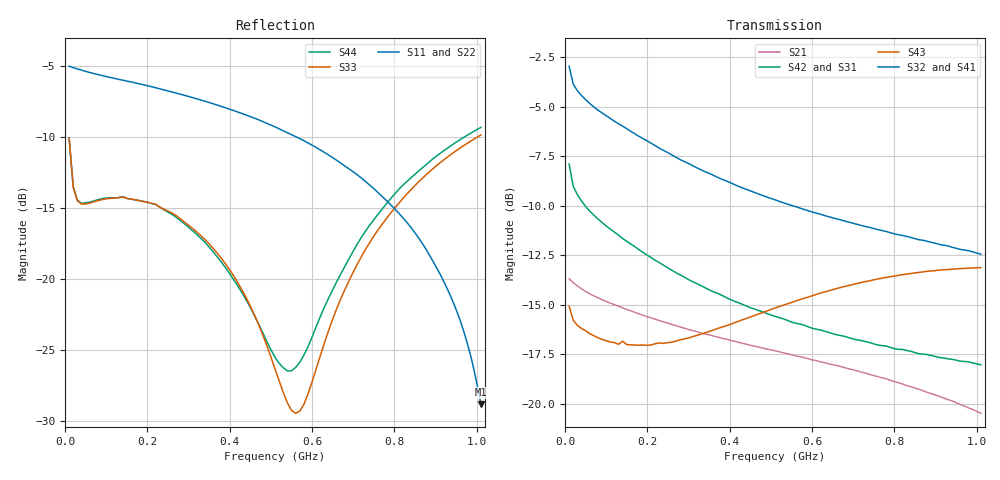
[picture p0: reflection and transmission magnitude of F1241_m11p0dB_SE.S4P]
! Integrated Device Technology
! Corporate Headquarters
! 6024 Silver Creek Valley Road
! San Jose, CA 95138  USA
! Phone:  1-408-284-8200
! Toll Free:  1-800-223-1366
! Webpage:  http://www.idt.com/
! Timing and RF Division
! 515 Groton Road, Suite 102
! Westford, MA 01886-6024
! Device:  F1241
! Description: Dual Intermediate Frequency Digital Variable Gain Amplifier
! Frequency:  10.0 -  500.00 MHz
! Package:  5x5 mm QFN Plastic Package: 32 pin
! Ports:  8 RF, 20 DC
!  Pin  1  = GA3  Pin 17  = RF OUT_B+
!  Pin  2  = GA4  Pin 18  = RF OUT_B-
!  Pin  3  = GA5  Pin 19  = STBY_B
!  Pin  4  = ISET_A  Pin 20  = Ground
!  Pin  5  = ISET_B  Pin 21  = Ground
!  Pin  6  = GB5  Pin 22  = STB_A
!  Pin  7  = GB4  Pin 23  = RF OUT_A-  = Port 4
!  Pin  8  = GB3  Pin 24  = RF OUT_A+  = Port 3
!  Pin  9  = GB2  Pin 25  = NO CONNECT
!  Pin 10  = GB1  Pin 26  = NO CONNECT
!  Pin 11  = RF IN_B+  Pin 27  = VCC
!  Pin 12  = RF IN_B-  Pin 28  = Ground
!  Pin 13  = Ground  Pin 29  = RF IN_A-  = Port 2
!  Pin 14  = VCC  Pin 30  = RF IN_A+  = Port 1
!  Pin 15  = NO CONNECT  Pin 31  = GA1
!  Pin 16  = NO CONNECT  Pin 32  = GA2
! State:  31
! Gain State:  -11.0 dB
! Voltages:  Vcc = +5.00 Volts  Icc approximately 160.0 mA or 80 mA per channel.
! Data:  The device was measured on a custom evaluation board which has
!  individual transmission lines to the RF pins.  Data was collected
!  using a calibrated network analyzer.  The evaluation board was
!  de-embedded using a port reference technique.
!  The reference plane is the edge of the package pin.
!  Only Channel A was measured.
!  This data is in single-ended operation.  If your needs are balanced
!  or differential S-parameters then this file needs to be used a
!  linear simulator.
! Misc:  Lot Code  160028MY
!  Action Tracker AT004
! Date Measured:  2014-08-14
! Date:  2014-08-28  MJV
! Note:
!  Integrated Device Technology supplies this data as a sample of measured
!  data at the package pin for this product.  Your particular data for this
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# Hz S dB R 50
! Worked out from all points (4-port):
!   101 points, 10 MHz to 1.01 GHz, reference 50 ohm
!   strongest paths, dB at 10 MHz, 260 MHz, 510 MHz, 760 MHz, 1.01 GHz:
!     S32: -2.9, -7.4, -9.7, -11.2, -12.4
!     S41: -2.9, -7.5, -9.8, -11.4, -12.7
!     S43: -15.1, -16.9, -15.2, -13.7, -13.1
!     S42: -7.9, -13.3, -15.6, -17.0, -18.0
!     S31: -7.9, -13.3, -15.7, -17.1, -18.0
!     S21: -13.7, -16.0, -17.3, -18.6, -20.5
!   lowest |S11| = -28.8 dB at 1.01 GHz (marker M1), VSWR 1.08, Z = 52.8 - j2.49 ohm
!   |S11| at or under -10 dB: 560.5 MHz to end of sweep
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1e7  -5.04 -3.5  -13.67 -7.3  -33.23 -2.9  -27.87 4.1
     -13.68 -7.2  -5.04 -3.4  -27.91 3.7  -33.23 -3.0
     -7.91 156.9  -2.94 164.1  -10.11 -46.3  -15.11 176.1
     -2.90 164.1  -7.89 157.0  -15.07 176.1  -10.07 -46.1
4e7  -5.32 -4.9  -14.17 -9.2  -34.09 -9.6  -28.31 -6.1
     -14.19 -9.2  -5.32 -4.8  -28.32 -5.8  -34.05 -9.7
     -9.76 156.4  -4.42 163.5  -14.74 -13.3  -16.25 166.5
     -4.38 163.3  -9.75 156.3  -16.19 166.5  -14.69 -12.9
3.7e8  -7.78 -15.9  -16.61 -31.4  -37.32 -11.5  -30.41 -16.6
       -16.62 -31.5  -7.76 -14.9  -30.24 -16.8  -37.34 -14.0
       -14.52 88.0  -8.55 121.9  -18.22 -7.3  -16.27 108.6
       -8.61 120.6  -14.42 87.3  -16.20 108.4  -18.47 -2.5
5.6e8  -9.99 -20.7  -17.54 -41.2  -37.23 -7.3  -30.49 -19.9
       -17.58 -41.3  -9.98 -19.5  -30.10 -20.8  -37.34 -10.2
       -16.02 60.2  -10.04 105.6  -29.47 57.0  -14.92 82.4
       -10.18 104.1  -15.93 58.5  -14.81 82.2  -26.25 67.9
7.1e8  -12.69 -25.0  -18.29 -49.2  -36.67 -6.3  -30.42 -24.1
       -18.34 -49.4  -12.75 -23.9  -29.73 -25.7  -36.70 -9.6
       -16.86 41.5  -10.94 93.8  -18.96 122.6  -14.05 63.2
       -11.14 92.3  -16.77 38.8  -13.92 63.1  -17.55 116.6
8.6e8  -17.18 -29.9  -19.23 -57.6  -35.73 -7.5  -30.32 -28.8
       -19.27 -57.7  -17.39 -30.0  -29.49 -31.3  -36.01 -10.3
       -17.52 25.1  -11.71 82.2  -13.14 124.3  -13.50 45.8
       -11.97 81.0  -17.47 21.7  -13.36 45.7  -12.39 120.5
1.01e9  -28.82 -40.6  -20.42 -66.4  -34.89 -11.1  -30.28 -34.4
        -20.48 -66.3  -29.04 -44.5  -29.29 -38.2  -35.07 -13.9
        -18.02 10.2  -12.44 70.7  -9.88 121.4  -13.26 30.1
        -12.73 69.9  -18.03 6.1  -13.12 30.1  -9.35 117.8
